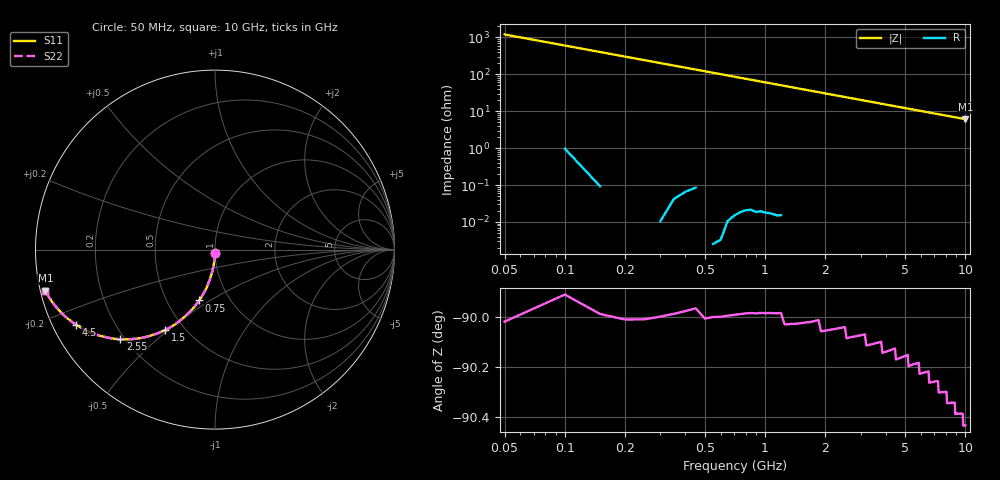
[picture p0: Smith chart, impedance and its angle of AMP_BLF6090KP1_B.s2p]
! Created Tue Sep  1 15:25:30 2009
# ghz S ma R 50
! 2 Port Network Data from SP1.SP block
! freq  magS11  angS11  magS21  angS21  magS12  angS12  magS22  angS22
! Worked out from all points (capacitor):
!   200 points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, 50 MHz to 10 GHz, reference 50 ohm
!   read as one part in shunt: C = 2.64 pF near 100 MHz
!   lowest |Z| = 6.09 ohm at 10 GHz (marker M1)
!   S11 on the Smith chart (normalised r, x): 50 MHz: 1.00, -0.04; 750 MHz: 0.72, -0.45; 1.5 GHz: 0.39, -0.49; 2.55 GHz: 0.18, -0.39; 4.5 GHz: 0.07, -0.25; 10 GHz: 0.01, -0.12
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0.05  0.02075 -91.1  0.9998 -1.2  0.9998 -1.2  0.02085 -91.1
0.1  0.04129 -92.4  0.9991 -2.4  0.9991 -2.4  0.04146 -92.5
0.15  0.06188 -93.6  0.998 -3.6  0.998 -3.6  0.06215 -93.6
0.2  0.08226 -94.7  0.9966 -4.7  0.9966 -4.7  0.08259 -94.7
0.25  0.1026 -95.9  0.9947 -5.9  0.9947 -5.9  0.103 -95.9
0.35  0.1429 -98.3  0.9896 -8.3  0.9896 -8.3  0.1434 -98.2
0.5  0.2033 -101.7  0.9792 -11.7  0.9792 -11.7  0.2025 -101.7
0.6  0.2416 -103.9  0.9704 -14.0  0.9704 -14.0  0.241 -104.0
0.75  0.2966 -107.3  0.9549 -17.3  0.9549 -17.3  0.2964 -107.3
0.9  0.3489 -110.5  0.9369 -20.4  0.9369 -20.4  0.349 -110.5
1.1  0.4137 -114.5  0.9101 -24.5  0.9101 -24.5  0.4141 -114.5
1.5  0.5273 -121.8  0.8497 -31.8  0.8497 -31.8  0.5271 -121.8
1.75  0.5859 -125.9  0.8101 -35.9  0.8101 -35.9  0.5862 -125.9
2.1  0.656 -131.0  0.7551 -41.0  0.7551 -41.0  0.6556 -131.0
2.55  0.7263 -136.5  0.6883 -46.6  0.6883 -46.6  0.7256 -136.5
3.4  0.8153 -144.6  0.5801 -54.7  0.5801 -54.7  0.815 -144.5
3.95  0.8534 -148.5  0.5227 -58.6  0.5227 -58.6  0.853 -148.5
4.5  0.8815 -151.7  0.4741 -61.9  0.4741 -61.9  0.881 -151.7
5.05  0.902 -154.4  0.4327 -64.6  0.4327 -64.6  0.9021 -154.4
6.7  0.9412 -160.1  0.3407 -70.4  0.3407 -70.4  0.9408 -160.1
8.35  0.9611 -163.8  0.2797 -74.1  0.2797 -74.1  0.9608 -163.8
10  0.9725 -166.4  0.2367 -76.8  0.2367 -76.8  0.9724 -166.3
